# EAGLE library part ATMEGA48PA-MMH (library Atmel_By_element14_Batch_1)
8-bit Microcontroller with In-System Programmable Flash
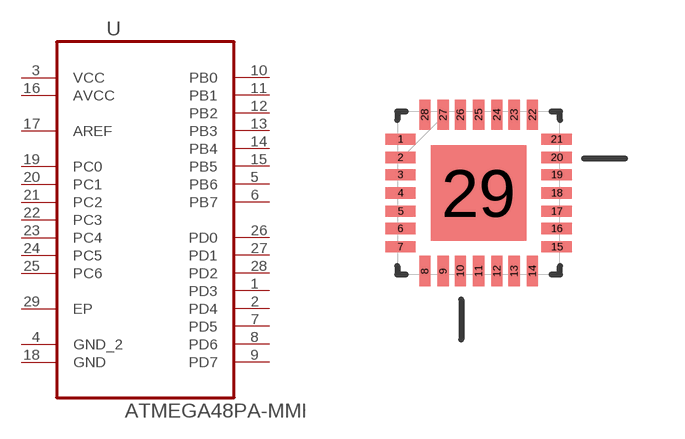
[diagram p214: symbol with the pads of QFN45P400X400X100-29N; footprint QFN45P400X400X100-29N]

Designator prefix U

## ATMEGA48PA-MMH (MPN: ATMEGA48PA-MMH; OC_FARNELL: 1748526; OC_NEWARK: 26R5634; PACKAGE: QFN-28; SUPPLIER: Atmel)  [QFN45P400X400X100-29N]
1  PD3
2  PD4
3  VCC  pwr
4  GND_2  pas
5  PB6
6  PB7
7  PD5
8  PD6
9  PD7
10  PB0
11  PB1
12  PB2
13  PB3
14  PB4
15  PB5
16  AVCC  pwr
17  AREF  in
18  GND  pas
19  PC0
20  PC1
21  PC2
22  PC3
23  PC4
24  PC5
25  PC6
26  PD0
27  PD1
28  PD2
29  EP  pas

## Footprint QFN45P400X400X100-29N (pad centres in mm)
smd 0.762 x 0.279: 1 -1.956,1.346; 2 -1.956,0.889; 3 -1.956,0.457; 4 -1.956,0; 5 -1.956,-0.457; 6 -1.956,-0.889; 7 -1.956,-1.346; 15 1.956,-1.346; 16 1.956,-0.889; 17 1.956,-0.457; 18 1.956,0; 19 1.956,0.457; 20 1.956,0.889; 21 1.956,1.346
smd 0.279 x 0.762: 8 -1.346,-1.956; 9 -0.889,-1.956; 10 -0.457,-1.956; 11 0,-1.956; 12 0.457,-1.956; 13 0.889,-1.956; 14 1.346,-1.956; 22 1.346,1.956; 23 0.889,1.956; 24 0.457,1.956; 25 0,1.956; 26 -0.457,1.956; 27 -0.889,1.956; 28 -1.346,1.956
smd 2.388 x 2.388: 29 0,0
